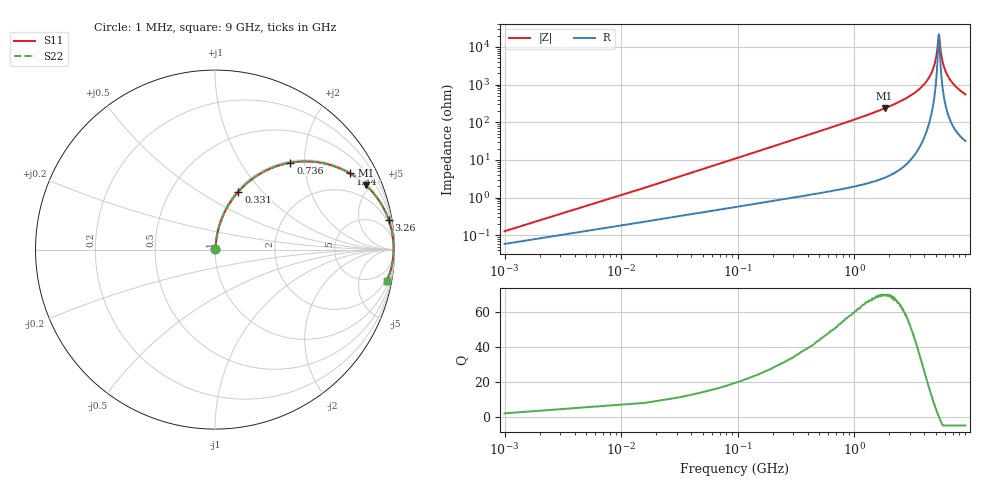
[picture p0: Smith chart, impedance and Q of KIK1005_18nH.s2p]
!version-3
!date-01.2023
!Series
# MHz S RI R 50
!Freq ReS11 ImS11 ReS21 ImS21 ReS12 ImS12 ReS22 ImS22
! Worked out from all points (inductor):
!   601 points, 1 MHz to 9 GHz, reference 50 ohm
!   read as one part in series: L = 18 nH near 46 MHz
!   highest Q = 69.6 at 1.82 GHz (marker M1), where L = 20.3 nH
!   self-resonance near 5.33 GHz
!   S11 on the Smith chart (normalised r, x): 1 MHz: 1.00, +0.00; 331 MHz: 1.02, +0.75; 736 MHz: 1.03, +1.70; 1.44 GHz: 1.05, +3.52; 3.26 GHz: 1, +12; 9 GHz: 2, -11
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1  0.000572 0.00113  0.9994 -0.00113  0.9994 -0.00113  0.000572 0.00113
61  0.00912 0.0681  0.9909 -0.0681  0.9909 -0.0681  0.00912 0.0681
91  0.0157 0.1008  0.9843 -0.1008  0.9843 -0.1008  0.0157 0.1008
181  0.0471 0.1938  0.9529 -0.1938  0.9529 -0.1938  0.0471 0.1938
331  0.1306 0.3233  0.8694 -0.3233  0.8694 -0.3233  0.1306 0.3233
736  0.4202 0.4842  0.5798 -0.4842  0.5798 -0.4842  0.4202 0.4842
1440  0.7524 0.4243  0.2476 -0.4243  0.2476 -0.4243  0.7524 0.4243
1520  0.7735 0.4113  0.2265 -0.4113  0.2265 -0.4113  0.7735 0.4113
1820  0.8402 0.3593  0.1598 -0.3593  0.1598 -0.3593  0.8402 0.3593
3020  0.9584 0.1903  0.0416 -0.1903  0.0416 -0.1903  0.9584 0.1903
3260  0.9684 0.1642  0.0316 -0.1642  0.0316 -0.1642  0.9684 0.1642
3980  0.9867 0.097  0.0133 -0.097  0.0133 -0.097  0.9867 0.097
4520  0.993 0.0546  0.00699 -0.0546  0.00699 -0.0546  0.993 0.0546
5000  0.9952 0.0213  0.0048 -0.0213  0.0048 -0.0213  0.9952 0.0213
5120  0.9954 0.0135  0.00463 -0.0135  0.00463 -0.0135  0.9954 0.0135
5280  0.9954 0.00307  0.00461 -0.00307  0.00461 -0.00307  0.9954 0.00307
5330  0.9954 0.000286  0.00464 -0.000286  0.00464 -0.000286  0.9954 0.000286
5640  0.9947 -0.0186  0.00532 0.0186  0.00532 0.0186  0.9947 -0.0186
6020  0.993 -0.0397  0.007 0.0397  0.007 0.0397  0.993 -0.0397
6630  0.9886 -0.0717  0.0114 0.0717  0.0114 0.0717  0.9886 -0.0717
7520  0.9794 -0.1129  0.0206 0.1129  0.0206 0.1129  0.9794 -0.1129
9000  0.9586 -0.1722  0.0414 0.1722  0.0414 0.1722  0.9586 -0.1722
